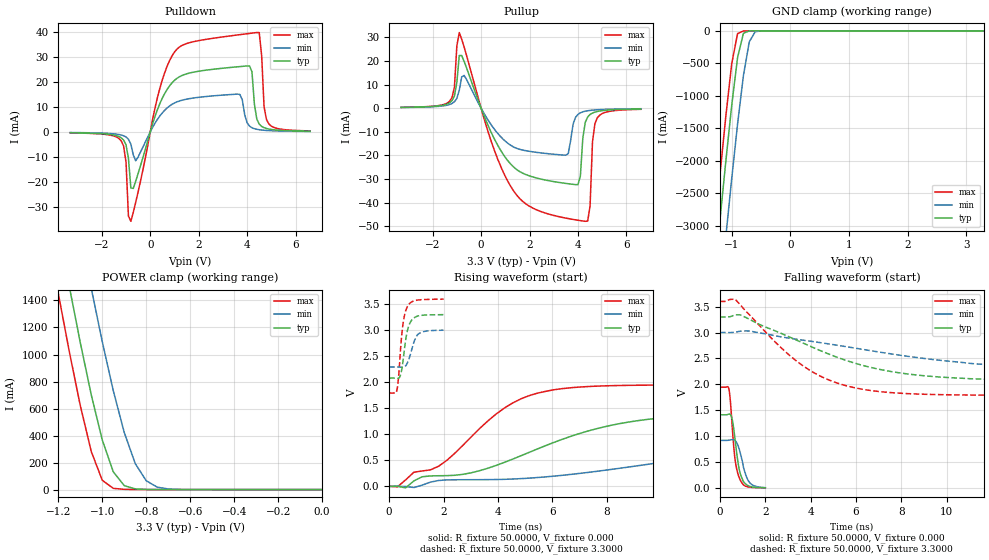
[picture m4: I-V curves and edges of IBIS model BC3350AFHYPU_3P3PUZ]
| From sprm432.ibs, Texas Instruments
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|   Model BC3350AFHYPU_3P3PUZ
[Model]   BC3350AFHYPU_3P3PUZ
Model_type   I/O
Polarity   Non-Inverting
Enable   Active-Low
Vinl =   0.9900V
Vinh =   2.3100V
Vmeas =   1.6500V
Cref =  15.0000pF
Rref = 100.0000M
Vref =  0.000V
C_comp   2.5478pF   2.6979pF   2.5389pF
[Temperature Range]   25.0000   0.1250k   -40.0000
[Voltage Range]   3.3000V   3.0000V   3.6000V
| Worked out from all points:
|   slope of the pulldown table from 0 to 0.495 V, typ, clamps not added: 36.7 ohm
|   slope of the pullup table from 0 to 0.495 V, typ, clamps not added: 41.5 ohm
|   GND clamp passes 1 mA (typ) near -0.68 V on its own axis
|   POWER clamp passes 1 mA (typ) near -0.78 V on its own axis
|   rising waveform, R_fixture 50.0000, V_fixture 0.000: 20-80 % time 4.63ns typ, 8.75ns min, 2.58ns max; typ from 0 V to 1.41 V
|   rising waveform, R_fixture 50.0000, V_fixture 3.3000: 20-80 % time 217ps typ, 267ps min, 191ps max; typ from 2.08 V to 3.29 V
|   falling waveform, R_fixture 50.0000, V_fixture 0.000: 20-80 % time 280ps typ, 337ps min, 246ps max; typ from 1.41 V to 0.006 V
|   falling waveform, R_fixture 50.0000, V_fixture 3.3000: 20-80 % time 4.41ns typ, 6.83ns min, 2.94ns max; typ from 3.3 V to 2.08 V
[Pulldown]
| voltage   I(typ)   I(min)   I(max)
-3.3V     -323uA     -232uA     -378uA
-1.2V     -2.324mA   -1.222mA   -3.542mA
-800mV    -22.43mA   -4.89mA    -35.82mA
-600mV    -19.72mA   -11.54mA   -28.19mA
300mV     9.041mA    5.104mA    13.91mA
1V        20.68mA    11.62mA    32.03mA
3.7V      26.21mA    15.05mA    39.01mA
4.1V      26.48mA    2.354mA    39.51mA
4.4V      5.156mA    1.069mA    39.85mA
4.5V      3.148mA    898.8uA    39.84mA
4.8V      1.388mA    604.9uA    4.95mA
6.6V      305uA      201uA      423uA
[Pullup]
| voltage   I(typ)   I(min)   I(max)
-3.3V     321uA      278uA      342uA
-1.3V     2.265mA    1.536mA    2.89mA
-900mV    22.26mA    7.57mA     31.99mA
600mV     -14.05mA   -9.585mA   -19.25mA
1.7V      -27.44mA   -17.71mA   -39.29mA
3.5V      -31.86mA   -19.91mA   -46.55mA
4V        -32.37mA   -2.653mA   -47.45mA
4.3V      -6.064mA   -1.298mA   -47.9mA
4.5V      -2.676mA   -959uA     -41.47mA
4.6V      -2.066mA   -847.2uA   -14.31mA
4.8V      -1.41mA    -686uA     -4.099mA
6.6V      -357uA     -250uA     -488uA
[GND_clamp]
| voltage   I(typ)   I(min)   I(max)
-3.3V     -23.37A    -24.46A    -22.74A
-1.3V     -3.836A    -5.005A    -3.135A
-1.2V     -2.907A    -4.075A    -2.207A
-1.1V     -2.003A    -3.163A    -1.312A
-1V       -1.147A    -2.276A    -506.4mA
-900mV    -411.6mA   -1.434A    -42.91mA
-800mV    -37.63mA   -687mA     -2.528mA
-700mV    -1.177mA   -169.1mA   -239.8uA
-600mV    -46.48uA   -14.64mA   -13.61uA
-400mV    -101.2nA   -50.84uA   -12.07nA
3.3V      257.9pA    366.9nA    239.1pA
[POWER_clamp]
| voltage   I(typ)   I(min)   I(max)
-3.3V     22.31A     23.05A     21.9A
-1.2V     1.938A     2.775A     1.451A
-1.15V    1.504A     2.334A     1.021A
-1.1V     1.087A     1.904A     621.5mA
-1.05V    700.4mA    1.489A     281.6mA
-1V       367mA      1.095A     69.05mA
-950mV    131.9mA    732.5mA    9.28mA
-900mV    29.16mA    422.1mA    1.919mA
-850mV    5.375mA    192.5mA    869.9uA
-800mV    1.306mA    65.55mA    473.6uA
-700mV    212.8uA    4.74mA     95.74uA
0V        257.9pA    1.786nA    301.7pA
[Ramp]
| variable   typ   min   max
dV/dt_r   0.7901/4.1464n   0.2800/7.1590n   1.1653/2.5286n
dV/dt_f   0.7010/4.0245n   0.3320/4.8901n   1.0798/2.8743n
R_load = 50.0000
[Rising Waveform]
R_fixture = 50.0000
V_fixture = 0.000
V_fixture_min = 0.000
V_fixture_max = 0.000
| time   V(typ)   V(min)   V(max)
0s        1.266nV    5.003nV    1.024nV
606.1ps   -29.56mV   -3.671mV   123.8mV
1.212ns   183mV      22.18mV    294.5mV
1.818ns   203mV      111.9mV    385.2mV
4.546ns   522.8mV    140mV      1.601V
6.364ns   901.8mV    211.2mV    1.875V
8.788ns   1.232V     369mV      1.937V
11.82ns   1.373V     585.9mV    1.945V
18.18ns   1.412V     849.2mV    1.945V
30ns      1.413V     917.5mV    1.945V
[Rising Waveform]
R_fixture = 50.0000
V_fixture = 3.3000
V_fixture_min = 3.0000
V_fixture_max = 3.6000
| time   V(typ)   V(min)   V(max)
0s        2.077V     2.29V      1.79V
282.8ps   2.073V     2.291V     1.839V
343.4ps   2.073V     2.29V      2.081V
404ps     2.116V     2.287V     2.518V
505.1ps   2.387V     2.284V     3.1V
606.1ps   2.806V     2.312V     3.365V
686.9ps   3.019V     2.387V     3.464V
828.3ps   3.188V     2.622V     3.539V
1.051ns   3.268V     2.911V     3.574V
2ns       3.293V     2.995V     3.592V
[Falling Waveform]
R_fixture = 50.0000
V_fixture = 0.000
V_fixture_min = 0.000
V_fixture_max = 0.000
| time   V(typ)   V(min)   V(max)
0s        1.413V     920.7mV    1.945V
404ps     1.428V     924.3mV    1.887V
464.6ps   1.415V     929.3mV    1.643V
525.3ps   1.35V      933.6mV    1.277V
646.5ps   1.004V     922.6mV    619.8mV
747.5ps   641.8mV    867.9mV    348.5mV
868.7ps   322.7mV    718.3mV    179.4mV
1.03ns    128.8mV    411.6mV    62.87mV
1.273ns   41.73mV    126.1mV    20.43mV
2ns       6.159mV    9.18mV     4.655mV
[Falling Waveform]
R_fixture = 50.0000
V_fixture = 3.3000
V_fixture_min = 3.0000
V_fixture_max = 3.6000
| time   V(typ)   V(min)   V(max)
0s        3.3V       3V         3.6V
666.7ps   3.34V      3.006V     3.644V
1.333ns   3.247V     3.027V     3.326V
2.667ns   2.989V     2.919V     2.719V
4ns       2.732V     2.832V     2.262V
5.111ns   2.532V     2.759V     2.034V
6.222ns   2.375V     2.68V      1.911V
8.222ns   2.204V     2.545V     1.823V
11.11ns   2.107V     2.401V     1.794V
22ns      2.077V     2.294V     1.79V
